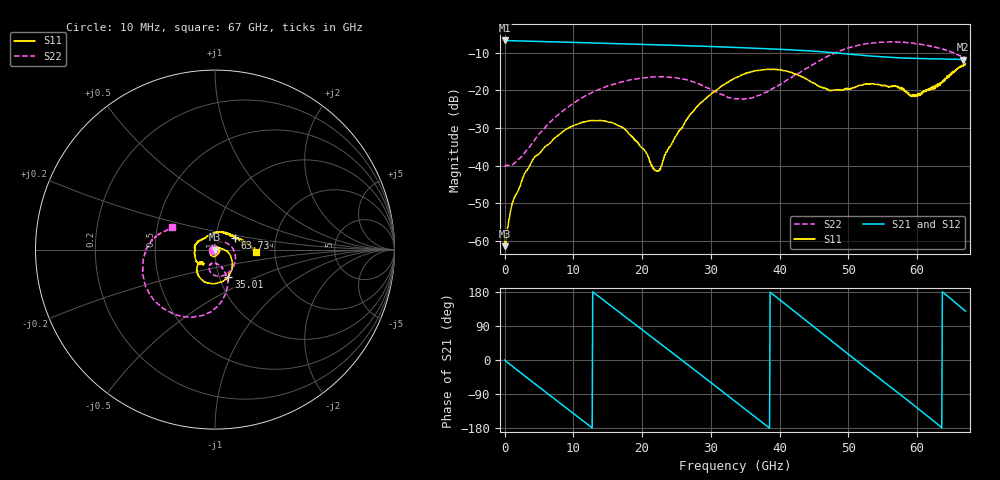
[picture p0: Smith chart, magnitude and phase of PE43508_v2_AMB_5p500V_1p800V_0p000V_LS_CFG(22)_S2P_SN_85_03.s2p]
!Keysight Technologies,N5227A,US51270237,A.10.43.00
!Date: Wednesday, August 22, 2018 17:08:50
!Correction: S11(Full 2 Port(1,3))
!S31(Full 2 Port(1,3))
!S13(Full 2 Port(1,3))
!S33(Full 2 Port(1,3))
!S2P File: Measurements: S11, S31, S13, S33:
# Hz S  dB  R 50
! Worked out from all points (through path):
!   801 points, 10 MHz to 67 GHz, reference 50 ohm
!   highest |S21| = -6.74 dB at 10 MHz (marker M1); lowest = -11.8 dB at 66.67 GHz (marker M2)
!   group delay of S21, straight-line fit = 39.2 ps
!   lowest |S11| = -61.4 dB at 93.74 MHz (marker M3), VSWR 1.00, Z = 50.1 + j0.0113 ohm
!   |S11| at or under -10 dB: start of sweep to end of sweep
!   |S22| runs from -40.3 to -7.1 dB; largest |S21 - S12| = 0.0031
!   S11 on the Smith chart (normalised r, x): 10 MHz: 1.00, -0.00; 35.01 GHz: 1.11, -0.34; 63.73 GHz: 1.24, +0.16; 67 GHz: 1.59, -0.05
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1e7  -59.32 -18.9  -6.74 -0.2  -6.74 -0.2  -40.27 -176.3
9.37375e7  -61.38 7.6  -6.75 -1.5  -6.76 -1.5  -40.03 179.4
1.3498e9  -48.75 21.4  -6.83 -19.6  -6.82 -19.6  -39.50 151.1
4.196875e9  -38.11 -14.0  -6.97 -59.8  -6.97 -59.8  -33.67 104.5
7.546375e9  -32.33 -51.1  -7.14 -106.8  -7.13 -106.7  -26.86 65.2
1.123082e10  -28.50 -89.4  -7.32 -158.1  -7.31 -158.1  -22.03 23.9
1.416164e10  -28.04 -118.5  -7.47 161.1  -7.46 161.2  -19.41 -4.4
1.74274e10  -30.24 -151.6  -7.65 115.8  -7.64 115.8  -17.57 -32.6
1.985579e10  -34.99 173.4  -7.78 82.1  -7.77 82.1  -16.73 -51.7
2.236791e10  -41.51 87.7  -7.92 47.2  -7.91 47.2  -16.40 -70.4
2.722469e10  -26.00 1.0  -8.18 -20.6  -8.18 -20.6  -17.61 -99.9
3.049045e10  -20.29 -23.8  -8.38 -66.4  -8.38 -66.4  -20.19 -109.5
3.3505e10  -16.74 -50.5  -8.58 -108.9  -8.58 -108.8  -22.21 -99.1
3.501228e10  -15.47 -63.7  -8.70 -130.2  -8.69 -130.0  -22.23 -87.9
3.95341e10  -14.47 -105.4  -9.06 165.8  -9.05 165.9  -19.10 -68.7
4.472582e10  -17.87 -138.9  -9.54 91.1  -9.52 91.2  -13.27 -71.2
5.016876e10  -19.68 -130.1  -10.37 12.5  -10.37 12.5  -8.62 -100.0
5.586291e10  -19.17 -177.9  -11.18 -67.6  -11.19 -68.0  -7.11 -139.1
5.979858e10  -21.12 112.9  -11.51 -123.3  -11.53 -123.6  -7.60 -164.8
6.373424e10  -17.84 30.4  -11.66 178.7  -11.73 178.5  -9.00 171.2
6.666505e10  -13.62 -0.0  -11.82 134.0  -11.89 134.4  -11.11 155.2
6.7e10  -12.84 -3.4  -11.81 128.8  -11.87 129.1  -11.33 152.8
